| IBIS file 70t3519z.ibs created by s2ibis2 version 1.1
| North Carolina State University Electronics Research Laboratory  1995
[IBIS ver]   2.1
[File name]   70t3519dr.ibs
[File Rev]   4.0
|1.0 : Original Version - Wei-Ling Chang
|2.0 : Corrected Ramp rates and package RLC values - Wei-Ling Chang
|3.0 : Replaced I/O and Input models with ADC models - Sunil Kashyap
|4.0 : Modified existing T3519 BF model for DR package - Trevor Hiatt
[Date]   01/20/04
[Source]   Integrated Device Technology, Inc.
[Notes]   1. Temperatures: typ=25C, min=70C, max=0C 2. Cmos125_2.5v
   process. 3. Ramp rates based on 50 ohm load.
[Copyright]   Copyright 2003, Integrated Device Technology, Inc. Integrated
   Device Technology, Inc. ("IDT") hereby grants the user of this
   IBIS model a non-exclusive, nontransferable license to use
   this IBIS model under the following terms. The user is granted
   this license only to use the IBIS model and is not granted
   rights to sell, copy (except as needed to run the IBIS model),
   rent, lease or sub-license the IBIS model in whole or in part,
   or in modified form to anyone. The User may modify the IBIS
   model to suit its specific applications, but rights to
   derivative works and such modifications shall belong to IDT.
   This IBIS model is provided on an AS IS" basis and IDT makes
   absolutely no warranty with respect to the information
   contained herein. IDT DISCLAIMS AND CUSTOMER WAIVES ALL
   WARRANTIES, EXPRESS AND IMPLIED, INCLUDING WARRANTIES OF
   MERCHANTABILITY AND FITNESS FOR A PARTICULAR PURPOSE. THE
   ENTIRE RISK AS TO QUALITY AND PERFORMANCE IS WITH THE USER
   ACCORDINGLY, IN NO EVENT SHALL IDT BE LIABLE FOR ANY DIRECT OR
   INDIRECT DAMAGES, WHETHER IN CONTRACT OR TORT, INCLUDING ANY
   LOST PROFITS OR OTHER INCIDENTAL, CONSEQUENTIAL, EXEMPLARY, OR
   PUNITIVE DAMAGES ARISING OUT OF THE USE OR APPLICATION OF THE
   IBIS model. Further, IDT reserves the right to make changes
   without notice to any product herein to improve reliability,
   function, or design. IDT does not convey any license under
   patent rights or any other intellectual property rights,
   including those of third parties. IDT is not obligated to
   provide maintenance or support for the licensed IBIS model.
|   Component 70t3519z
[Component]   70t3519z
[Manufacturer]   Integrated Device Technology
[Package]   TQFP (DR208)
| variable   typ   min   max
R_pkg   0.16   0.13   0.19
L_pkg   4.82nH   3.56nH   6.07nH
C_pkg   1.47pF   1.28pF   1.66pF
| NOTE:
| The model_name inpad25, inpadzz25, inpadbs25, and iopad25 work for
| both 3.3v and 2.5v vddq.  When vddq is 3.3v, the model names are
| inpad33, inpadzz33, inpadbs33, and iopad33.  When vddq is 2.5v,
| the model names will be inpad25, inpadzz25, inpadbs25,and iopad25.
[Pin]  signal_name   model_name   R_pin   L_pin   C_pin
1   io19l   iopad25
2   io19r   iopad25
3   io20l   iopad25
4   io20r   iopad25
5   VDDQL   POWER
6   vss   GND
7   io21l   iopad25
8   io21r   iopad25
9   io22l   iopad25
10   io22r   iopad25
11   VDDQR   POWER
12   vss   GND
13   io23l   iopad25
14   io23r   iopad25
15   io24l   iopad25
16   io24r   iopad25
17   VDDQL   POWER
18   vss   GND
19   io25l   iopad25
20   io25r   iopad25
21   io26l   iopad25
22   io26r   iopad25
23   VDDQR   POWER
24   zzr   inpadzz25
25   VDD   POWER
26   VDD   POWER
27   vss   GND
28   vss   GND
29   VDDQL   POWER
30   vss   GND
31   io27r   iopad25
32   io27l   iopad25
33   io28r   iopad25
34   io28l   iopad25
35   VDDQR   POWER
36   vss   GND
37   io29r   iopad25
38   io29l   iopad25
39   io30r   iopad25
40   io30l   iopad25
41   VDDQL   POWER
42   vss   GND
43   io31r   iopad25
44   io31l   iopad25
45   io32r   iopad25
46   io32l   iopad25
47   VDDQR   POWER
48   vss   GND
49   io33r   iopad25
50   io33l   iopad25
51   io34r   iopad25
52   io34l   iopad25
53   vss   GND
54   VDDQL   POWER
55   io35r   iopad25
56   io35l   iopad25
57   plftr#   inpad25
59   colr#   iopad25
60   intr#   iopad25
63   a17r   inpad25
64   a16r   inpad25
65   a15r   inpad25
66   a14r   inpad25
67   a13r   inpad25
68   a12r   inpad25
69   a11r   inpad25
70   a10r   inpad25
71   a9r   inpad25
72   a8r   inpad25
73   a7r   inpad25
74   be3r#   inpad25
75   be2r#   inpad25
76   be1r#   inpad25
77   be0r#   inpad25
78   ce1r   inpad25
79   ce0r   inpad25
80   VDD   POWER
81   VDD   POWER
82   vss   GND
83   vss   GND
84   clkr   inpad25
85   oer#   inpad25
86   rwr#   inpad25
87   adsr#   inpad25
88   cntenr#   inpad25
89   repeatr#   inpad25
90   a6r   inpad25
91   a5r   inpad25
92   a4r   inpad25
93   a3r   inpad25
94   a2r   inpad25
95   a1r   inpad25
96   a0r   inpad25
97   VDD   POWER
98   vss   GND
100   optr   inpad25
101   io0l   iopad25
102   io0r   iopad25
103   VDDQL   POWER
104   vss   GND
105   io1l   iopad25
106   io1r   iopad25
107   io2l   iopad25
108   io2r   iopad25
109   VDDQR   POWER
110   vss   GND
111   io3l   iopad25
112   io3r   iopad25
113   io4l   iopad25
114   io4r   iopad25
115   VDDQL   POWER
116   vss   GND
117   io5l   iopad25
118   io5r   iopad25
119   io6l   iopad25
120   io6r   iopad25
121   VDDQR   POWER
122   vss   GND
123   io7l   iopad25
124   io7r   iopad25
125   io8l   iopad25
126   io8r   iopad25
127   VDDQL   POWER
128   zzl   inpadzz25
129   vss   GND
130   vss   GND
131   VDD   POWER
132   VDD   POWER
133   VDDQR   POWER
134   vss   GND
135   io9r   iopad25
136   io9l   iopad25
137   io10r   iopad25
138   io10l   iopad25
139   VDDQL   POWER
140   vss   GND
141   io11r   iopad25
142   io11l   iopad25
143   io12r   iopad25
144   io12l   iopad25
145   VDDQR   POWER
146   vss   GND
147   io13r   iopad25
148   io13l   iopad25
149   io14r   iopad25
150   io14l   iopad25
151   VDDQL   POWER
152   vss   GND
153   io15r   iopad25
154   io15l   iopad25
155   io16r   iopad25
156   io16l   iopad25
157   vss   GND
158   VDDQR   POWER
159   io17r   iopad25
160   io17l   iopad25
161   optl   inpad25
163   VDD   POWER
164   VDD   POWER
165   a0l   inpad25
166   a1l   inpad25
167   a2l   inpad25
168   a3l   inpad25
169   a4l   inpad25
170   a5l   inpad25
171   a6l   inpad25
172   repeatl#   inpad25
173   cntenl#   inpad25
174   adsl#   inpad25
175   rwl#   inpad25
176   oel#   inpad25
177   clkl   inpad25
178   vss   GND
179   vss   GND
180   VDD   POWER
181   VDD   POWER
182   ce0l#   inpad25
183   ce1l   inpad25
184   be0l#   inpad25
185   be1l#   inpad25
186   be2l#   inpad25
187   be3l#   inpad25
188   a7l   inpad25
189   a8l   inpad25
190   a9l   inpad25
191   a10l   inpad25
192   a11l   inpad25
193   a12l   inpad25
194   a13l   inpad25
195   a14l   inpad25
196   a15l   inpad25
197   a16l   inpad25
198   a17l   inpad25
201   intl#   iopad25
202   coll#   iopad25
203   plftl#   inpad25
204   vss   GND
205   io18l   iopad25
206   io18r   iopad25
207   VDDQR   POWER
208   vss   GND
| NDAIN NDAIN   dummy_model
| OC   OC   dummy_model
| PUD   PUD   dummy_model|
[Pin Mapping]  pulldown_ref   pullup_ref
1   vss   vddql
2   vss   vddqr
3   vss   vddql
4   vss   vddqr
5   nc   vddql
6   vss   nc
7   vss   vddql
8   vss   vddqr
9   vss   vddql
10   vss   vddqr
11   nc   vddqr
12   vss   nc
13   vss   vddql
14   vss   vddqr
15   vss   vddql
16   vss   vddqr
17   nc   vddql
18   vss   nc
19   vss   vddql
20   vss   vddqr
21   vss   vddql
22   vss   vddqr
23   nc   vddqr
24   vss   vdd
25   nc   vdd
26   nc   vdd
27   vss   nc
28   vss   nc
29   nc   vddql
30   vss   nc
31   vss   vddqr
32   vss   vddql
33   vss   vddqr
34   vss   vddql
35   nc   vddqr
36   vss   nc
37   vss   vddqr
38   vss   vddql
39   vss   vddqr
40   vss   vddql
41   nc   vddql
42   vss   nc
43   vss   vddqr
44   vss   vddql
45   vss   vddqr
46   vss   vddql
47   nc   vddqr
48   vss   nc
49   vss   vddqr
50   vss   vddql
51   vss   vddqr
52   vss   vddql
53   vss   nc
54   nc   vddql
55   vss   vddqr
56   vss   vddql
57   vss   vdd
59   vss   vddqr
60   vss   vddqr
63   vss   vdd
64   vss   vdd
65   vss   vdd
66   vss   vdd
67   vss   vdd
68   vss   vdd
69   vss   vdd
70   vss   vdd
71   vss   vdd
72   vss   vdd
73   vss   vdd
74   vss   vdd
75   vss   vdd
76   vss   vdd
77   vss   vdd
78   vss   vdd
79   vss   vdd
80   nc   vdd
81   nc   vdd
82   vss   nc
83   vss   nc
84   vss   vddqr
85   vss   vdd
86   vss   vdd
87   vss   vddqr
88   vss   vddqr
89   vss   vddqr
90   vss   vdd
91   vss   vdd
92   vss   vdd
93   vss   vdd
94   vss   vdd
95   vss   vdd
96   vss   vdd
97   nc   vdd
98   vss   nc
100   vss   vdd
101   vss   vddql
102   vss   vddqr
103   nc   vddql
104   vss   nc
105   vss   vddql
106   vss   vddqr
107   vss   vddql
108   vss   vddqr
109   nc   vddqr
110   vss   nc
111   vss   vddql
112   vss   vddqr
113   vss   vddql
114   vss   vddqr
115   nc   vddql
116   vss   nc
117   vss   vddql
118   vss   vddqr
119   vss   vddql
120   vss   vddqr
121   nc   vddqr
122   vss   nc
123   vss   vddql
124   vss   vddqr
125   vss   vddql
126   vss   vddqr
127   nc   vddql
128   vss   vdd
129   vss   nc
130   vss   nc
131   nc   vdd
132   nc   vdd
133   nc   vddqr
134   vss   nc
135   vss   vddqr
136   vss   vddql
137   vss   vddqr
138   vss   vddql
139   nc   vddql
140   vss   nc
141   vss   vddqr
142   vss   vddql
143   vss   vddqr
144   vss   vddql
145   nc   vddqr
146   vss   nc
147   vss   vddqr
148   vss   vddql
149   vss   vddqr
150   vss   vddql
151   nc   vddql
152   vss   nc
153   vss   vddqr
154   vss   vddql
155   vss   vddqr
156   vss   vddql
157   vss   nc
158   nc   vddqr
159   vss   vddqr
160   vss   vddql
161   vss   vdd
163   nc   vdd
164   nc   vdd
165   vss   vdd
166   vss   vdd
167   vss   vdd
168   vss   vdd
169   vss   vdd
170   vss   vdd
171   vss   vdd
172   vss   vddql
173   vss   vddql
174   vss   vddql
175   vss   vdd
176   vss   vdd
177   vss   vddql
178   vss   nc
179   vss   nc
180   nc   vdd
181   nc   vdd
182   vss   vdd
183   vss   vdd
184   vss   vdd
185   vss   vdd
186   vss   vdd
187   vss   vdd
188   vss   vdd
189   vss   vdd
190   vss   vdd
191   vss   vdd
192   vss   vdd
193   vss   vdd
194   vss   vdd
195   vss   vdd
196   vss   vdd
197   vss   vdd
198   vss   vdd
201   vss   vddql
202   vss   vddql
203   vss   vddql
204   vss   nc
205   vss   vddql
206   vss   vddqr
207   nc   vddqr
208   vss   nc
| Models and submodels in the file (8): inpad25 (Input), inpad33 (Input), inpadzz25 (Input), inpadzz33 (Input), inpadbs25 (Input), inpadbs33 (Input), iopad25 (I/O), iopad33 (I/O)
